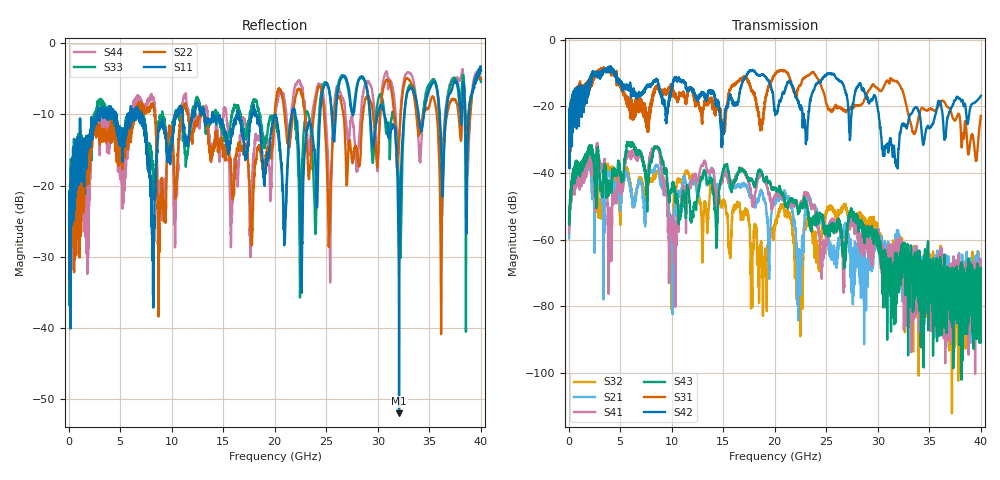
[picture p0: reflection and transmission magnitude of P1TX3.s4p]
!Agilent Technologies,N5245A,MY49151084,A.09.20.08
!Agilent N5245A: A.09.20.08
!Date: Thursday, March 01, 2012 14:16:46
!Correction: S11(Full 4 Port(1,2,3,4))
!S12(Full 4 Port(1,2,3,4))
!S13(Full 4 Port(1,2,3,4))
!S14(Full 4 Port(1,2,3,4))
!S21(Full 4 Port(1,2,3,4))
!S22(Full 4 Port(1,2,3,4))
!S23(Full 4 Port(1,2,3,4))
!S24(Full 4 Port(1,2,3,4))
!S31(Full 4 Port(1,2,3,4))
!S32(Full 4 Port(1,2,3,4))
!S33(Full 4 Port(1,2,3,4))
!S34(Full 4 Port(1,2,3,4))
!S41(Full 4 Port(1,2,3,4))
!S42(Full 4 Port(1,2,3,4))
!S43(Full 4 Port(1,2,3,4))
!S44(Full 4 Port(1,2,3,4))
!S4P File: Measurements: <S11,S12,S13,S14>,
!<S21,S22,S23,S24>,
!<S31,S32,S33,S34>,
!<S41,S42,S43,S44>:
# Hz S  dB  R 50
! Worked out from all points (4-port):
!   3996 points, 50 MHz to 40 GHz, reference 50 ohm
!   strongest paths, dB at 50 MHz, 10.04 GHz, 20.03 GHz, 30.02 GHz, 40 GHz:
!     S42: -23.6, -13.7, -22.0, -21.4, -16.8
!     S31: -25.2, -14.0, -10.4, -14.8, -22.9
!     S43: -55.1, -44.7, -44.6, -60.9, -78.5
!     S41: -57.9, -56.7, -46.7, -59.1, -73.2
!     S21: -59.7, -61.0, -49.1, -57.9, -71.8
!     S32: -55.4, -69.1, -55.1, -57.2, -73.8
!   lowest |S11| = -52.0 dB at 32.06 GHz (marker M1), VSWR 1.01, Z = 49.9 - j0.235 ohm
!   |S11| at or under -10 dB: start of sweep to 2.739 GHz; 7.082 GHz to 10.35 GHz (3.268 GHz wide, 37.5 % of centre); 18.22 GHz to 21.67 GHz (3.453 GHz wide, 17.3 % of centre)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
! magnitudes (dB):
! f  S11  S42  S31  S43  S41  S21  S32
! 50 MHz  -24.0  -23.6  -25.2  -55.1  -57.9  -59.7  -55.4
! 8.51 GHz  -16.6  -11.7  -13.8  -32.5  -32.2  -37.8  -40.3
! 10.35 GHz  -10.0  -11.9  -16.2  -47.4  -63.2  -48.9  -44.5
! 13.15 GHz  -9.8  -16.7  -19.3  -39.6  -36.5  -39.1  -49.9
! 22.36 GHz  -16.7  -19.6  -13.8  -51.8  -51.8  -62.8  -67.6
! 32.06 GHz  -52.0  -31.3  -13.4  -75.2  -65.0  -58.3  -62.3
! 40 GHz  -3.9  -16.8  -22.9  -78.5  -73.2  -71.8  -73.8
